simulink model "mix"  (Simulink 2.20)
settings: Solver=ode45  StartTime=0.0  StopTime=10000  RelTol=1e-3  AbsTol=1e-6
undefined symbols (not defined in the file or in its folder): Automatic

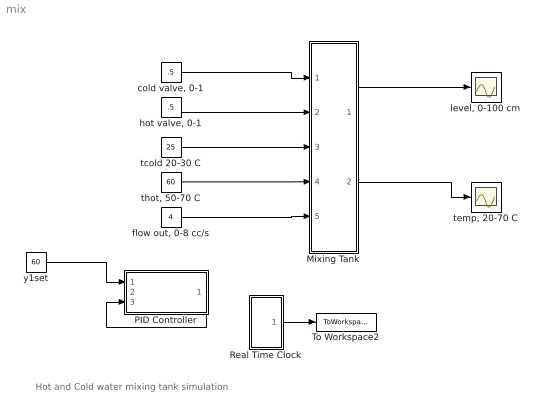
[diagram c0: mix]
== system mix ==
  note: Hot and Cold water mixing tank simulation
  Mixing Tank : Subsystem  mask{Ts=1, tinit=40, fcmax=4, fhmax=4, hmax=100, A=3, hinit=50}
      mask prompts: Ts "Sample Time, Ts, sec"; tinit "Initial temp, tinit deg C"; fcmax "Max cold flow, fcmax, cc/sec"; fhmax "Max hot flow, fhmax. cc/sec"; hmax "Tank height, hmax, cm"; A "Area of Tank, cm2"; hinit "Inital level in tank, cm"
  PID Controller : Subsystem  mask(Real PID Controller){am_flag=Automatic, co=.5, Ts=1, Kc=.1, taui=5, taud=0, co_max=1, co_min=0, al=0}
      mask prompts: am_flag "Auto/Manual Switch"; co "Manual Controller Output"; Ts "Sample Time,Ts"; Kc "Kc: Proportional Gain: Negative for DIRECT Action"; taui "taui: Integral time"; taud "Derivative Time, taud"; co_max "Upper limit for controller output"; co_min "Lower limit for controller output"; al "Noise filter tim const, al"
      mask help: Programmed by Babu Joseph, Washington Universtiy in St. Louis, 1998
  Real Time Clock : Subsystem  mask(Sample time){Ts=1}
      mask prompts: Ts "Sample time"
      mask help: This block is used to set the sample time.
  To Workspace2 : ToWorkspace  VariableName=t  SampleTime=1
  "cold valve, 0-1" : Constant  Value=.5
  "flow out, 0-8 cc/s" : Constant  Value=4
  "hot valve, 0-1" : Constant  Value=.5
  "level, 0-100 cm" : Scope
  tcold 20-30 C : Constant  Value=25
  "temp, 20-70 C" : Scope
  "thot, 50-70 C" : Constant  Value=60
  y1set : Constant  Value=60
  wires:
  y1set/1 -> PID Controller/1(setpt)
  PID Controller/1(output) -> PID Controller/3(out_fdbk)
  "cold valve, 0-1"/1 -> Mixing Tank/1(xc)
  "hot valve, 0-1"/1 -> Mixing Tank/2(xh)
  tcold 20-30 C/1 -> Mixing Tank/3(tc)
  "thot, 50-70 C"/1 -> Mixing Tank/4(th)
  "flow out, 0-8 cc/s"/1 -> Mixing Tank/5(fout)
  Mixing Tank/1(h) -> "level, 0-100 cm"/1
  Mixing Tank/2(t) -> "temp, 20-70 C"/1
  Real Time Clock/1("Clock ") -> To Workspace2/1

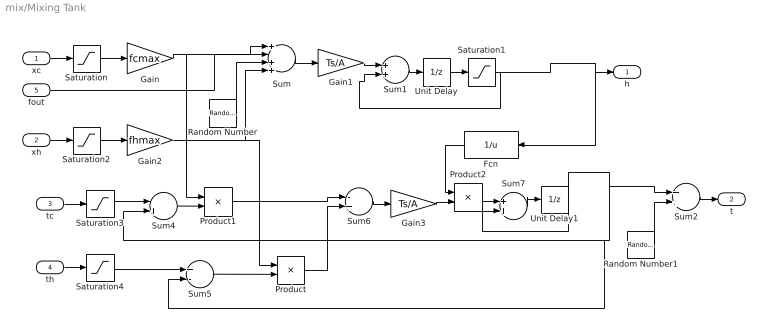
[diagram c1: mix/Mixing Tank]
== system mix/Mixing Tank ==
  xc : Inport  Port=1  PortWidth=-1  SampleTime=-1
  xh : Inport  Port=2  PortWidth=-1  SampleTime=-1
  tc : Inport  Port=3  PortWidth=-1  SampleTime=-1
  th : Inport  Port=4  PortWidth=-1  SampleTime=-1
  fout : Inport  Port=5  PortWidth=-1  SampleTime=-1
  Fcn : Fcn  Orientation=left  Expr=1/u
  Gain : Gain  Gain=fcmax
  Gain1 : Gain  Gain=Ts/A
  Gain2 : Gain  Gain=fhmax
  Gain3 : Gain  Gain=Ts/A
  Product : Product  Inputs=2
  Product1 : Product  Inputs=2
  Product2 : Product  Inputs=2
  Random Number : RandomNumber  Mean=0  Variance=.02  Seed=0  SampleTime=0
  Random Number1 : RandomNumber  Mean=0  Variance=.2  Seed=0  SampleTime=0
  Saturation : Saturate  UpperLimit=1  LowerLimit=0
  Saturation1 : Saturate  UpperLimit=hmax  LowerLimit=10
  Saturation2 : Saturate  UpperLimit=1  LowerLimit=0
  Saturation3 : Saturate  UpperLimit=30  LowerLimit=20
  Saturation4 : Saturate  UpperLimit=70  LowerLimit=50
  Sum : Sum  Inputs=+-++
  Sum1 : Sum  Inputs=++
  Sum2 : Sum  Inputs=++
  Sum4 : Sum  Inputs=-+
  Sum5 : Sum  Inputs=+-
  Sum6 : Sum  Inputs=-+
  Sum7 : Sum  Inputs=++
  Unit Delay : UnitDelay  X0=hinit  SampleTime=Ts
  Unit Delay1 : UnitDelay  X0=tinit  SampleTime=Ts
  h : Outport  Port=1  InitialOutput=0
  t : Outport  Port=2  InitialOutput=0
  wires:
  fout/1 -> Sum/2
  Sum/1 -> Gain1/1
  Gain1/1 -> Sum1/1
  Sum1/1 -> Unit Delay/1
  Unit Delay/1 -> Saturation1/1
  Saturation1/1 -> Sum1/2, h/1, Fcn/1
  Saturation2/1 -> Gain2/1
  xh/1 -> Saturation2/1
  Saturation/1 -> Gain/1
  xc/1 -> Saturation/1
  Saturation3/1 -> Sum4/1
  tc/1 -> Saturation3/1
  Saturation4/1 -> Sum5/1
  th/1 -> Saturation4/1
  Sum4/1 -> Product1/2
  Gain/1 -> Sum/1, Product1/1
  Sum5/1 -> Product/2
  Product1/1 -> Sum6/1
  Product/1 -> Sum6/2
  Sum6/1 -> Gain3/1
  Gain3/1 -> Product2/2
  Fcn/1 -> Product2/1
  Product2/1 -> Sum7/1
  Unit Delay1/1 -> Sum7/2, Sum5/2, Sum4/2, Sum2/1
  Sum7/1 -> Unit Delay1/1
  Gain2/1 -> Product/1, Sum/4
  Random Number/1 -> Sum/3
  Random Number1/1 -> Sum2/2
  Sum2/1 -> t/1

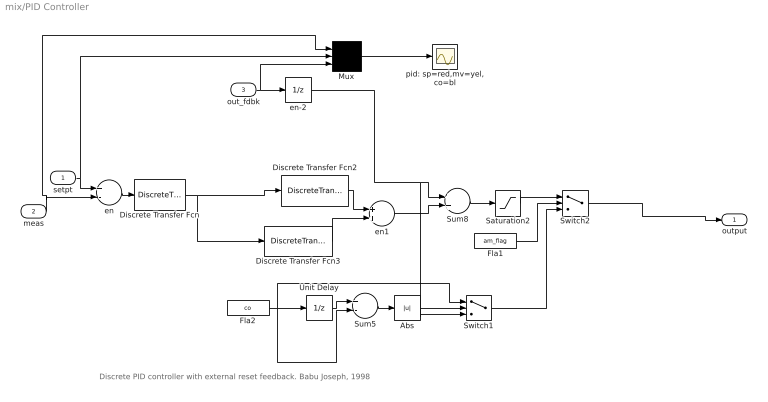
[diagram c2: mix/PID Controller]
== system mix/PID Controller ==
  note: Discrete PID controller with external reset feedback. Babu Joseph, 1998
  setpt : Inport  Port=1  PortWidth=-1  SampleTime=-1
  meas : Inport  Port=2  PortWidth=-1  SampleTime=-1
  out_fdbk : Inport  Port=3  PortWidth=-1  SampleTime=-1
  Abs : Abs
  Discrete Transfer Fcn : DiscreteTransferFcn  Numerator="[Ts   0]"  Denominator="[(al+Ts)  -al]"  SampleTime=Ts
  Discrete Transfer Fcn2 : DiscreteTransferFcn  Numerator="Kc*[ (1+Ts/taui)  -1 ]"  Denominator="[ 1  0 ]"  SampleTime=Ts
  Discrete Transfer Fcn3 : DiscreteTransferFcn  Numerator=Kc*taud*[1 -2 1]  Denominator=[ 1 0 0]  SampleTime=Ts
  Fla1 : Constant  Value=am_flag
  Fla2 : Constant  Value=co
  Mux : Mux  Inputs=3
  Saturation2 : Saturate  UpperLimit=co_max  LowerLimit=co_min
  Sum5 : Sum  Inputs=+-
  Sum8 : Sum  Inputs=++
  Switch1 : Switch  Threshold=0.0001
  Switch2 : Switch  Threshold=1.5
  Unit Delay : UnitDelay  X0=0  SampleTime=Ts
  en : Sum  Inputs=+-
  en-2 : UnitDelay  X0=co  SampleTime=Ts
  en1 : Sum  Inputs=++
  pid: sp=red,mv=yel,co=bl : Scope
  output : Outport  Port=1  InitialOutput=0
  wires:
  Discrete Transfer Fcn/1 -> Discrete Transfer Fcn3/1, Discrete Transfer Fcn2/1
  en/1 -> Discrete Transfer Fcn/1
  setpt/1 -> Mux/2, en/1
  en1/1 -> Sum8/2
  Discrete Transfer Fcn2/1 -> en1/1
  Discrete Transfer Fcn3/1 -> en1/2
  Switch2/1 -> output/1
  en-2/1 -> Switch1/3, Sum8/1
  Switch1/1 -> Switch2/3
  Unit Delay/1 -> Sum5/1
  Fla2/1 -> Unit Delay/1, Sum5/2, Switch1/1
  Sum5/1 -> Abs/1
  Abs/1 -> Switch1/2
  Fla1/1 -> Switch2/2
  Saturation2/1 -> Switch2/1
  Sum8/1 -> Saturation2/1
  meas/1 -> en/2, Mux/1
  out_fdbk/1 -> en-2/1, Mux/3
  Mux/1 -> pid: sp=red,mv=yel,co=bl/1

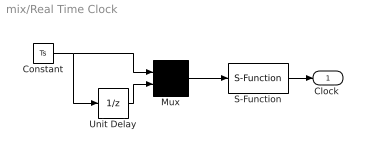
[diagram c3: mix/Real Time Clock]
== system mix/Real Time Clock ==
  Constant : Constant  Value=Ts
  Mux : Mux  Inputs=2
  S-Function : S-Function  FunctionName=wait3  PortCounts=[]  SFunctionModules=''
  Unit Delay : UnitDelay  X0=0  SampleTime=Ts
  "Clock " : Outport  Port=1  InitialOutput=0
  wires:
  S-Function/1 -> "Clock "/1
  Mux/1 -> S-Function/1
  Unit Delay/1 -> Mux/2
  Constant/1 -> Mux/1, Unit Delay/1
